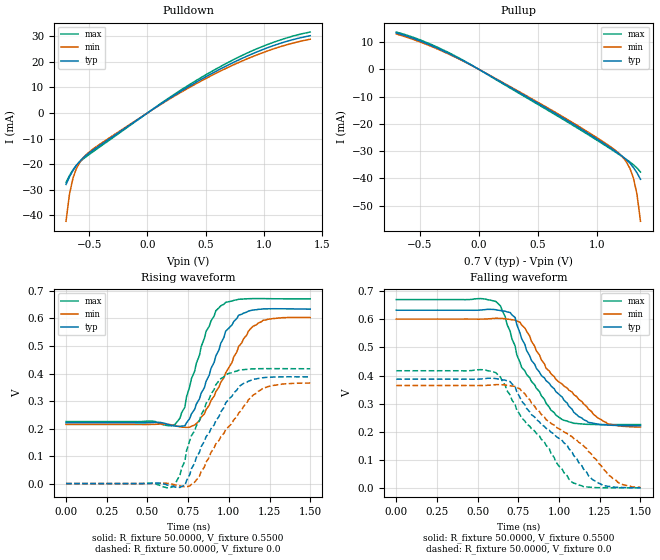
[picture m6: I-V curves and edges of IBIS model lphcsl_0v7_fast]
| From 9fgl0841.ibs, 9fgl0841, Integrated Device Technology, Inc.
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[Model]   lphcsl_0v7_fast
Model_type Output
Polarity   Non-Inverting
Enable   Active-High
Vmeas =  0.4000V
Cref =   2.0000pF
Rref =   0.0
Vref =   0.4000V
C_comp   1.1000pF   1.0000pF   1.2000pF
[Temperature Range]   25.0000   85.0000   -40.0000
[Voltage Range]   0.7000V   0.6700V   0.7400V
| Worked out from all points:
|   slope of the pulldown table from 0 to 0.105 V, typ, clamps not added: 32.9 ohm
|   slope of the pullup table from 0 to 0.105 V, typ, clamps not added: 40.5 ohm
|   rising waveform, R_fixture 50.0000, V_fixture 0.5500: 20-80 % time 164ps typ, 205ps min, 146ps max; typ from 0.221 V to 0.634 V
|   rising waveform, R_fixture 50.0000, V_fixture 0.0: 20-80 % time 214ps typ, 252ps min, 170ps max; typ from 0 V to 0.388 V
|   falling waveform, R_fixture 50.0000, V_fixture 0.5500: 20-80 % time 286ps typ, 333ps min, 230ps max; typ from 0.633 V to 0.221 V
|   falling waveform, R_fixture 50.0000, V_fixture 0.0: 20-80 % time 372ps typ, 416ps min, 296ps max; typ from 0.387 V to 0 V
[Pulldown]
|Voltage   I(typ)   I(min)   I(max)
-700mV    -27.91mA   -42.29mA   -27.13mA
-670mV    -24.93mA   -31.58mA   -24.4mA
-640mV    -22.46mA   -25.38mA   -22.16mA
-610mV    -20.43mA   -21.63mA   -20.41mA
-550mV    -17.42mA   -17.37mA   -17.87mA
-460mV    -14.27mA   -13.81mA   -14.87mA
170mV     5.111mA    4.867mA    5.413mA
620mV     17mA       16.18mA    17.92mA
830mV     21.65mA    20.59mA    22.8mA
1.01V     25.07mA    23.84mA    26.32mA
1.22V     28.24mA    26.89mA    29.6mA
1.4V      30.17mA    28.8mA     31.59mA
[Pullup]
|Voltage   I(typ)   I(min)   I(max)
-700mV    13.37mA    12.97mA    13.69mA
-400mV    8.685mA    8.356mA    9.067mA
-40mV     976.3uA    932.1uA    1.037mA
710mV     -17.77mA   -17.34mA   -18.25mA
1.01V     -25.83mA   -25.34mA   -26.25mA
1.16V     -30.15mA   -29.81mA   -30.44mA
1.22V     -32.05mA   -32.24mA   -32.17mA
1.25V     -33.15mA   -33.95mA   -33.06mA
1.28V     -34.44mA   -36.32mA   -33.98mA
1.31V     -36.02mA   -39.87mA   -35mA
1.34V     -37.97mA   -45.72mA   -36.19mA
1.37V     -40.34mA   -55.75mA   -37.7mA
[Ramp]
| variable   typ   min   max
dV/dt_r  0.2327/0.2120n   0.2192/0.2438n   0.2503/0.1864n
dV/dt_f  0.2497/0.2565n   0.2337/0.2967n   0.2701/0.2197n
R_load = 50.0000
[Rising Waveform]
R_fixture= 50.0000
V_fixture= 0.5500
V_fixture_min= 0.5200
V_fixture_max= 0.5800
|time   V(typ)   V(min)   V(max)
0s        221mV      214.9mV    225.3mV
650ps     210.9mV    212.4mV    210.2mV
730ps     209.9mV    204.6mV    278mV
800ps     288.3mV    217.9mV    436.5mV
860ps     371.3mV    269.2mV    553.3mV
950ps     508.9mV    368mV      645.7mV
1.06ns    611.8mV    498mV      669.8mV
1.15ns    630.9mV    572mV      672.2mV
1.24ns    635.1mV    597mV      672mV
1.5ns     634mV      603.5mV    671mV
[Rising Waveform]
R_fixture= 50.0000
V_fixture= 0.0
V_fixture_min= 0.0
V_fixture_max= 0.0
|time   V(typ)   V(min)   V(max)
0s        0V         0V         0V
640ps     -8.091mV   -315uV     -15.03mV
670ps     -12.45mV   -4.428mV   -2.669mV
730ps     -7.069mV   -11.24mV   81.56mV
770ps     53.48mV    -3.061mV   174.1mV
860ps     170.1mV    77.73mV    291.3mV
980ps     292.4mV    195mV      395.2mV
1.09ns    363.9mV    280.3mV    414.1mV
1.21ns    384.8mV    347.2mV    417.7mV
1.5ns     387.8mV    365.3mV    417.2mV
[Falling Waveform]
R_fixture= 50.0000
V_fixture= 0.5500
V_fixture_min= 0.5200
V_fixture_max= 0.5800
|time   V(typ)   V(min)   V(max)
0s        632.9mV    601.2mV    670.7mV
610ps     634.7mV    604mV      664.5mV
640ps     631.8mV    603.8mV    648.2mV
730ps     606.8mV    597.8mV    505.4mV
770ps     531.2mV    580.1mV    429.2mV
830ps     454.4mV    522.4mV    379.2mV
950ps     363mV      406.2mV    276.6mV
1.12ns    254.1mV    315.7mV    228.3mV
1.3ns     223.5mV    227.5mV    225.4mV
1.5ns     221.4mV    216.3mV    225.3mV
[Falling Waveform]
R_fixture= 50.0000
V_fixture= 0.0
V_fixture_min= 0.0
V_fixture_max= 0.0
|time   V(typ)   V(min)   V(max)
0s        387.1mV    364.6mV    417.1mV
610ps     389.4mV    367.5mV    410.7mV
730ps     361.1mV    361.3mV    296.8mV
830ps     261mV      302.3mV    210.9mV
920ps     212mV      242.7mV    151.3mV
1.08ns    127mV      182.3mV    19.84mV
1.18ns    43.36mV    129.4mV    2.496mV
1.27ns    7.62mV     67.37mV    132.2uV
1.38ns    1.242mV    13.5mV     -120.3uV
1.5ns     113.4uV    1.53mV     -45.16uV
